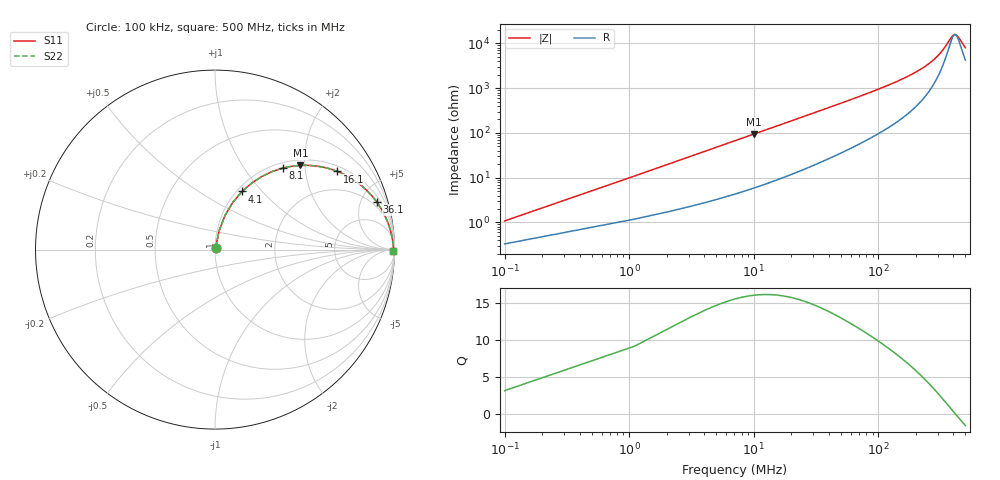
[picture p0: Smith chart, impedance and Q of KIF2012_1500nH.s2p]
!version-2
!date-12.2020
!Series
# MHz S RI R 50
!Freq ReS11 ImS11 ReS21 ImS21 ReS12 ImS12 ReS22 ImS22
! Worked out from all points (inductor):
!   501 points, 100 kHz to 500 MHz, reference 50 ohm
!   read as one part in series: L = 1.53 uH near 2.1 MHz
!   highest Q = 16 at 10.1 MHz (marker M1), where L = 1.49 uH
!   self-resonance near 412.8 MHz
!   S11 on the Smith chart (normalised r, x): 100 kHz: 1.01, +0.02; 4.1 MHz: 1.06, +0.78; 8.1 MHz: 1.10, +1.53; 16.1 MHz: 1.19, +2.99; 36.1 MHz: 1.47, +6.63; 500 MHz: open
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0.1  0.00341 0.0102  0.9966 -0.0102  0.9966 -0.0102  0.00341 0.0102
1.1  0.0228 0.1042  0.9772 -0.1042  0.9772 -0.1042  0.0228 0.1042
3.1  0.0988 0.2625  0.9012 -0.2625  0.9012 -0.2625  0.0988 0.2625
4.1  0.1505 0.3237  0.8495 -0.3237  0.8495 -0.3237  0.1505 0.3237
6.1  0.2647 0.4095  0.7353 -0.4095  0.7353 -0.4095  0.2647 0.4095
8.1  0.3766 0.4539  0.6234 -0.4539  0.6234 -0.4539  0.3766 0.4539
10.1  0.4755 0.4692  0.5245 -0.4692  0.5245 -0.4692  0.4755 0.4692
13.1  0.5943 0.461  0.4057 -0.461  0.4057 -0.461  0.5943 0.461
16.1  0.6816 0.4357  0.3184 -0.4357  0.3184 -0.4357  0.6816 0.4357
24.1  0.817 0.3554  0.183 -0.3554  0.183 -0.3554  0.817 0.3554
36.1  0.9014 0.265  0.0986 -0.265  0.0986 -0.265  0.9014 0.265
57.1  0.9519 0.1776  0.0481 -0.1776  0.0481 -0.1776  0.9519 0.1776
84.1  0.973 0.1218  0.027 -0.1218  0.027 -0.1218  0.973 0.1218
119.1  0.9833 0.0838  0.0167 -0.0838  0.0167 -0.0838  0.9833 0.0838
167.1  0.9889 0.0552  0.0111 -0.0552  0.0111 -0.0552  0.9889 0.0552
250.1  0.9924 0.0282  0.00755 -0.0282  0.00755 -0.0282  0.9924 0.0282
334.1  0.9936 0.0116  0.00643 -0.0116  0.00643 -0.0116  0.9936 0.0116
390.1  0.9937 0.00308  0.00626 -0.00308  0.00626 -0.00308  0.9937 0.00308
404.1  0.9937 0.00116  0.00626 -0.00116  0.00626 -0.00116  0.9937 0.00116
417.1  0.9937 -0.000558  0.00627 0.000558  0.00627 0.000558  0.9937 -0.000558
437.1  0.9937 -0.00311  0.00632 0.00311  0.00632 0.00311  0.9937 -0.00311
500  0.9934 -0.0105  0.00664 0.0105  0.00664 0.0105  0.9934 -0.0105
